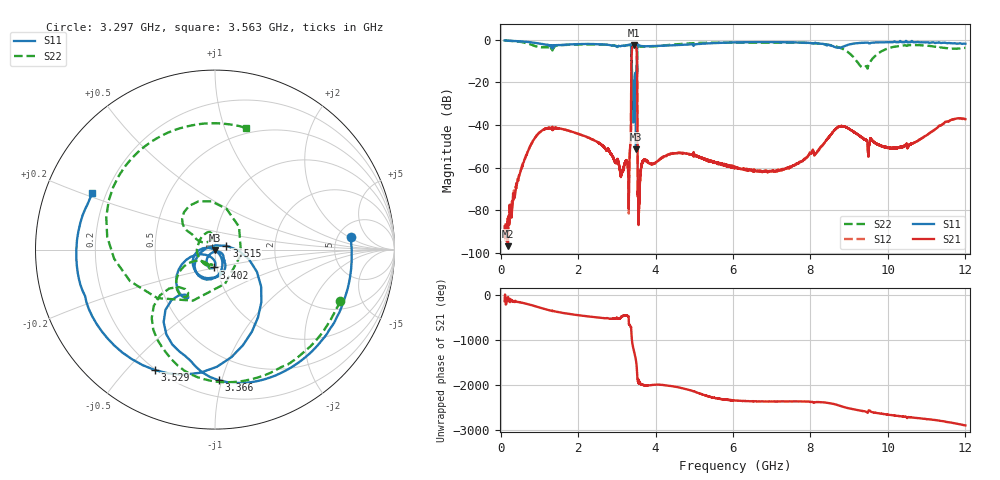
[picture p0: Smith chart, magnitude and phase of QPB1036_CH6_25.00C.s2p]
! TDS: K:\Engsetup\Winsaw\QPB1036_ALL
! Channel 1
! Ports=1 2
! seg 1=100.000000 1100.000000 101
! seg 2=1101.000000 1501.000000 401
! seg 3=1502.000000 2502.000000 101
! seg 4=2503.000000 3803.000000 1301
! seg 5=3804.000000 5004.000000 121
! seg 6=5005.000000 6005.000000 1001
! seg 7=6006.000000 8406.000000 241
! seg 8=8407.000000 10607.000000 2201
! seg 9=10608.000000 12008.000000 141
! Points=5609
! FailCode=0
! Topology=ALL_SE(12)
!VNA Cal loaded =QPB1036_ALL_25C
!PS1(V)= 5.000
!PS(mA)= 0.700
!PS2(V)= 1.170
!PS(mA)= -0.100
!PS3(V)= 1.170
!PS(mA)= 0.100
!PS4(V)= 0.630
!PS(mA)= -0.100
!Temp (C)= 25.00
# MHz S DB R 50
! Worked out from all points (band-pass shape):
!   5609 points, 100 MHz to 12.01 GHz, reference 50 ohm
!   highest |S21| = -2.63 dB at 3.436 GHz (marker M1); lowest = -97.0 dB at 180 MHz (marker M2)
!   |S21| within 3 dB of the highest: 3.386 GHz to 3.516 GHz (130 MHz wide, 3.77 % of centre)
!   lowest |S11| = -51.5 dB at 3.495 GHz (marker M3), VSWR 1.01, Z = 49.8 - j0.163 ohm
!   |S11| at or under -10 dB: 3.378338 GHz to 3.382041 GHz (3.703 MHz wide, 0.11 % of centre); 3.383 GHz to 3.519 GHz (135.5 MHz wide, 3.93 % of centre)
!   |S22| runs from -25.1 to -0.3 dB; largest |S21 - S12| = 0.0068
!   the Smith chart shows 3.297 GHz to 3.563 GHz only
!   S11 on the Smith chart (normalised r, x): 3.297 GHz: 6.52, +2.21; 3.366 GHz: 0.32, -0.98; 3.402 GHz: 0.97, -0.20; 3.515 GHz: 1.14, +0.05; 3.529 GHz: 0.20, -0.60; 3.563 GHz: 0.15, +0.21
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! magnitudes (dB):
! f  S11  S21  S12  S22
! 100 MHz  -0.3  -87.7  -91.8  -0.3
! 180 MHz  -0.4  -97.0  -86.8  -0.4
! 1.124 GHz  -2.2  -41.9  -42.0  -3.5
! 2.092 GHz  -2.0  -44.8  -44.7  -2.2
! 3.248 GHz  -2.6  -56.6  -56.9  -2.5
! 3.297 GHz  -2.4  -64.6  -63.6  -2.5
! 3.334 GHz  -2.2  -53.2  -53.6  -2.4
! 3.366 GHz  -2.8  -40.3  -40.3  -3.0
! 3.402 GHz  -20.0  -3.4  -3.4  -19.7
! 3.436 GHz  -24.1  -2.6  -2.6  -20.0
! 3.495 GHz  -51.5  -3.3  -3.2  -24.9
! 3.515 GHz  -23.4  -5.2  -5.2  -12.8
! 3.529 GHz  -2.5  -29.4  -29.4  -4.4
! 3.563 GHz  -2.5  -82.5  -75.8  -3.1
! 3.675 GHz  -3.0  -57.1  -56.9  -3.2
! 4.074 GHz  -2.8  -56.6  -56.6  -2.9
! 6.056 GHz  -1.2  -59.5  -59.7  -1.3
! 8.046 GHz  -1.5  -53.0  -52.9  -1.5
! 8.791 GHz  -3.6  -40.5  -40.6  -3.9
! 9.369 GHz  -1.4  -46.5  -46.4  -13.0
! 10.02 GHz  -1.1  -50.6  -50.7  -3.9
! 12.01 GHz  -1.8  -37.3  -37.2  -3.8
